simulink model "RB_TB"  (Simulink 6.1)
settings: Solver=ode3  SolverMode=SingleTasking  StartTime=0  StopTime=0.1  FixedStep=0.01  RelTol=1e-3
libraries: simulink x2
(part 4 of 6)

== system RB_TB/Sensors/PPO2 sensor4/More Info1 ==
  note: Terminology:
  note: Sensor fusion by using a sliding observer for an underwater breathing system Salvatore Carotenuto, Luigi Iannelli, Sabato Manfredi, Stefania Santini e-mail: luigi.iannelli@unisannio.it, {salcarot, smanfred, stsantin}@unina.it ... When working in critical conditions or environments, such as under the sea, the control-loop has to be fault-tolerant. In other words the control strategy of the rebreather system has to be 'robust' against sensor failures. An error on the actual oxygen level measurement, especially in the set point proximity, can cause a disease to the diver and may have fatal consequences. Thus, in the counterlung control-loop some hardware redundancy is desired: usually the system output (oxygen partial pressure) is measured through three sensors so that eventual sensor faults can be detected and isolated for the diver safety. Of course, by introducing this redundancy, an algorithm that decides which measurement value to give to the controller is needed. The problem of designing this algorithm is called 'sensor fusion' problem. ... The performance of the proposed strategy are discussed comparing it with a more traditional approach based on a decision by majority criteria [7], [8], usually named as voting logic, which is currently implemented in some commercial rebreathers and is a proven technology in some applicative areas as fly-by-wire control [9].

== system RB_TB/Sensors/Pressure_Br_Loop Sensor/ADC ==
  note: This subsystem models a typical 15-bit analog-to-digital converter having an input range of 0-3 volts
  note: Model: RB_TB/Sensors/Pressure_ambient Sensor/ADC
  voltage : Inport  Port=1  LatchInput=off
  limit : Saturate  UpperLimit=2^15  LowerLimit=0
  quantize : Quantizer  QuantizationInterval=1
  scale : Gain  Gain=2^15/3
  pcm : Outport
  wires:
  voltage/1 -> scale/1
  quantize/1 -> limit/1
  scale/1 -> quantize/1
  limit/1 -> pcm/1

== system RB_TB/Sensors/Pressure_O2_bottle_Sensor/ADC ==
  note: Model: RB_TB/Sensors/Pressure_ambient Sensor/ADC
  note: This subsystem models a typical 15-bit analog-to-digital converter having an input range of 0-3 volts
  voltage : Inport  Port=1  LatchInput=off
  limit : Saturate  UpperLimit=2^15  LowerLimit=0
  quantize : Quantizer  QuantizationInterval=1
  scale : Gain  Gain=2^15/3
  pcm : Outport
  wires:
  limit/1 -> pcm/1
  scale/1 -> quantize/1
  quantize/1 -> limit/1
  voltage/1 -> scale/1

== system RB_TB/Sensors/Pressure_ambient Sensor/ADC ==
  note: Model: RB_TB/Sensors/Pressure_ambient Sensor/ADC
  note: This subsystem models a typical 15-bit analog-to-digital converter having an input range of 0-3 volts
  voltage : Inport  Port=1  LatchInput=off
  limit : Saturate  UpperLimit=2^15  LowerLimit=0
  quantize : Quantizer  QuantizationInterval=1
  scale : Gain  Gain=2^15/3
  pcm : Outport
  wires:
  limit/1 -> pcm/1
  scale/1 -> quantize/1
  quantize/1 -> limit/1
  voltage/1 -> scale/1

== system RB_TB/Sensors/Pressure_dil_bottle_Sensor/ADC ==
  note: This subsystem models a typical 15-bit analog-to-digital converter having an input range of 0-3 volts
  note: Model: RB_TB/Sensors/Pressure_ambient Sensor/ADC
  voltage : Inport  Port=1  LatchInput=off
  limit : Saturate  UpperLimit=2^15  LowerLimit=0
  quantize : Quantizer  QuantizationInterval=1
  scale : Gain  Gain=2^15/3
  pcm : Outport
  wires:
  voltage/1 -> scale/1
  quantize/1 -> limit/1
  scale/1 -> quantize/1
  limit/1 -> pcm/1

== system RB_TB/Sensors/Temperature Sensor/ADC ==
  note: This subsystem models a typical 16-bit analog-to-digital converter having an input range of 0-5 volts
  note: Model: RB_TB/Sensors/temperature_sensor/ADC
  voltage : Inport  Port=1  LatchInput=off
  limit : Saturate  UpperLimit=65535  LowerLimit=0
  quantize : Quantizer  QuantizationInterval=1
  scale : Gain  Gain=65536/5
  pcm : Outport
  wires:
  voltage/1 -> scale/1
  quantize/1 -> limit/1
  scale/1 -> quantize/1
  limit/1 -> pcm/1

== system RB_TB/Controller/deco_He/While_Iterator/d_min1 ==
  note: Model: RB_TB/Controller/deco_He/While_Iterator/d_minX
  Pt_new : Inport  Port=1  LatchInput=off
  In1 : Inport  Port=2  LatchInput=off
  In2 : Inport  Port=3  LatchInput=off
  BC : BusCreator  DialogController=Simulink.DDGSource_Bus
  BS1 : BusSelector  DialogController=Simulink.DDGSource_Bus  OutputSignals=He_b,M0,He_k,Pt
  BS2 : BusSelector  DialogController=Simulink.DDGSource_Bus  OutputSignals=rate_asc,asc_time,while,cnc_He,Palv_next,Palv
  Mux2 : Mux  Inputs=6
  Product2 : Product
  Sum1 : Sum  Inputs=-+|
  Switch : Switch  Threshold=2
  Switch1 : Switch  Threshold=2
  fnc : Fcn  Expr=u(6)-u(5)*u(2)*(u(3)-1/u(1))-(u(6)-u(4)+u(5)*u(2)/u(1))*exp(-u(1)*u(3))
  prod : Gain  Gain=10
  bus1 : Outport
  d_min : Outport  Port=2
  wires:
  BS2/1 -> Mux2/2  "<rate_asc>"
  In2/1 -> BS2/1
  BS2/5 -> Switch1/1  "<Palv_next>"
  BS2/3 -> Switch1/2, Switch/2  "<while>"
  BS2/6 -> Switch1/3  "<Palv>"
  Switch1/1 -> Mux2/6
  Pt_new/1 -> Switch/1
  BS1/4 -> Switch/3  "<Pt>"
  Switch/1 -> Mux2/4, Sum1/2  "Pt"
  BC/1 -> bus1/1
  Product2/1 -> d_min/1
  prod/1 -> Product2/1
  Sum1/1 -> Product2/2
  In1/1 -> BS1/1
  BS2/4 -> Mux2/5  "<cnc_He>"
  BS2/2 -> Mux2/3  "<asc_time>"
  fnc/1 -> BC/4  "Pt_stop"
  Mux2/1 -> fnc/1
  BS1/2 -> BC/2, Sum1/1  "<M0>"
  BS1/1 -> BC/1, prod/1  "<He_b>"
  BS1/3 -> BC/3, Mux2/1  "<He_k>"

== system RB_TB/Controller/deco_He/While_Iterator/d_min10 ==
  note: Model: RB_TB/Controller/deco_He/While_Iterator/d_minX
  Pt_new : Inport  Port=1  LatchInput=off
  In1 : Inport  Port=2  LatchInput=off
  In2 : Inport  Port=3  LatchInput=off
  BC : BusCreator  DialogController=Simulink.DDGSource_Bus
  BS1 : BusSelector  DialogController=Simulink.DDGSource_Bus  OutputSignals=He_b,M0,He_k,Pt
  BS2 : BusSelector  DialogController=Simulink.DDGSource_Bus  OutputSignals=rate_asc,asc_time,while,cnc_He,Palv_next,Palv
  Mux2 : Mux  Inputs=6
  Product2 : Product
  Sum1 : Sum  Inputs=-+|
  Switch : Switch  Threshold=2
  Switch1 : Switch  Threshold=2
  fnc : Fcn  Expr=u(6)-u(5)*u(2)*(u(3)-1/u(1))-(u(6)-u(4)+u(5)*u(2)/u(1))*exp(-u(1)*u(3))
  prod : Gain  Gain=10
  bus1 : Outport
  d_min : Outport  Port=2
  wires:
  BS1/3 -> Mux2/1, BC/3  "<He_k>"
  BS1/1 -> prod/1, BC/1  "<He_b>"
  BS1/2 -> Sum1/1, BC/2  "<M0>"
  Mux2/1 -> fnc/1
  fnc/1 -> BC/4  "Pt_stop"
  BS2/2 -> Mux2/3  "<asc_time>"
  BS2/4 -> Mux2/5  "<cnc_He>"
  In1/1 -> BS1/1
  Sum1/1 -> Product2/2
  prod/1 -> Product2/1
  Product2/1 -> d_min/1
  BC/1 -> bus1/1
  Switch/1 -> Sum1/2, Mux2/4  "Pt"
  BS1/4 -> Switch/3  "<Pt>"
  Pt_new/1 -> Switch/1
  Switch1/1 -> Mux2/6
  BS2/6 -> Switch1/3  "<Palv>"
  BS2/3 -> Switch/2, Switch1/2  "<while>"
  BS2/5 -> Switch1/1  "<Palv_next>"
  In2/1 -> BS2/1
  BS2/1 -> Mux2/2  "<rate_asc>"

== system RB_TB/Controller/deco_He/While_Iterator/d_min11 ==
  note: Model: RB_TB/Controller/deco_He/While_Iterator/d_minX
  Pt_new : Inport  Port=1  LatchInput=off
  In1 : Inport  Port=2  LatchInput=off
  In2 : Inport  Port=3  LatchInput=off
  BC : BusCreator  DialogController=Simulink.DDGSource_Bus
  BS1 : BusSelector  DialogController=Simulink.DDGSource_Bus  OutputSignals=He_b,M0,He_k,Pt
  BS2 : BusSelector  DialogController=Simulink.DDGSource_Bus  OutputSignals=rate_asc,asc_time,while,cnc_He,Palv_next,Palv
  Mux2 : Mux  Inputs=6
  Product2 : Product
  Sum1 : Sum  Inputs=-+|
  Switch : Switch  Threshold=2
  Switch1 : Switch  Threshold=2
  fnc : Fcn  Expr=u(6)-u(5)*u(2)*(u(3)-1/u(1))-(u(6)-u(4)+u(5)*u(2)/u(1))*exp(-u(1)*u(3))
  prod : Gain  Gain=10
  bus1 : Outport
  d_min : Outport  Port=2
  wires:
  BS2/1 -> Mux2/2  "<rate_asc>"
  In2/1 -> BS2/1
  BS2/5 -> Switch1/1  "<Palv_next>"
  BS2/3 -> Switch1/2, Switch/2  "<while>"
  BS2/6 -> Switch1/3  "<Palv>"
  Switch1/1 -> Mux2/6
  Pt_new/1 -> Switch/1
  BS1/4 -> Switch/3  "<Pt>"
  Switch/1 -> Mux2/4, Sum1/2  "Pt"
  BC/1 -> bus1/1
  Product2/1 -> d_min/1
  prod/1 -> Product2/1
  Sum1/1 -> Product2/2
  In1/1 -> BS1/1
  BS2/4 -> Mux2/5  "<cnc_He>"
  BS2/2 -> Mux2/3  "<asc_time>"
  fnc/1 -> BC/4  "Pt_stop"
  Mux2/1 -> fnc/1
  BS1/2 -> BC/2, Sum1/1  "<M0>"
  BS1/1 -> BC/1, prod/1  "<He_b>"
  BS1/3 -> BC/3, Mux2/1  "<He_k>"

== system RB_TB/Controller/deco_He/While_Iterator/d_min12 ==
  note: Model: RB_TB/Controller/deco_He/While_Iterator/d_minX
  Pt_new : Inport  Port=1  LatchInput=off
  In1 : Inport  Port=2  LatchInput=off
  In2 : Inport  Port=3  LatchInput=off
  BC : BusCreator  DialogController=Simulink.DDGSource_Bus
  BS1 : BusSelector  DialogController=Simulink.DDGSource_Bus  OutputSignals=He_b,M0,He_k,Pt
  BS2 : BusSelector  DialogController=Simulink.DDGSource_Bus  OutputSignals=rate_asc,asc_time,while,cnc_He,Palv_next,Palv
  Mux2 : Mux  Inputs=6
  Product2 : Product
  Sum1 : Sum  Inputs=-+|
  Switch : Switch  Threshold=2
  Switch1 : Switch  Threshold=2
  fnc : Fcn  Expr=u(6)-u(5)*u(2)*(u(3)-1/u(1))-(u(6)-u(4)+u(5)*u(2)/u(1))*exp(-u(1)*u(3))
  prod : Gain  Gain=10
  bus1 : Outport
  d_min : Outport  Port=2
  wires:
  BS1/3 -> Mux2/1, BC/3  "<He_k>"
  BS1/1 -> prod/1, BC/1  "<He_b>"
  BS1/2 -> Sum1/1, BC/2  "<M0>"
  Mux2/1 -> fnc/1
  fnc/1 -> BC/4  "Pt_stop"
  BS2/2 -> Mux2/3  "<asc_time>"
  BS2/4 -> Mux2/5  "<cnc_He>"
  In1/1 -> BS1/1
  Sum1/1 -> Product2/2
  prod/1 -> Product2/1
  Product2/1 -> d_min/1
  BC/1 -> bus1/1
  Switch/1 -> Sum1/2, Mux2/4  "Pt"
  BS1/4 -> Switch/3  "<Pt>"
  Pt_new/1 -> Switch/1
  Switch1/1 -> Mux2/6
  BS2/6 -> Switch1/3  "<Palv>"
  BS2/3 -> Switch/2, Switch1/2  "<while>"
  BS2/5 -> Switch1/1  "<Palv_next>"
  In2/1 -> BS2/1
  BS2/1 -> Mux2/2  "<rate_asc>"

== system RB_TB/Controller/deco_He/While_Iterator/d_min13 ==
  note: Model: RB_TB/Controller/deco_He/While_Iterator/d_minX
  Pt_new : Inport  Port=1  LatchInput=off
  In1 : Inport  Port=2  LatchInput=off
  In2 : Inport  Port=3  LatchInput=off
  BC : BusCreator  DialogController=Simulink.DDGSource_Bus
  BS1 : BusSelector  DialogController=Simulink.DDGSource_Bus  OutputSignals=He_b,M0,He_k,Pt
  BS2 : BusSelector  DialogController=Simulink.DDGSource_Bus  OutputSignals=rate_asc,asc_time,while,cnc_He,Palv_next,Palv
  Mux2 : Mux  Inputs=6
  Product2 : Product
  Sum1 : Sum  Inputs=-+|
  Switch : Switch  Threshold=2
  Switch1 : Switch  Threshold=2
  fnc : Fcn  Expr=u(6)-u(5)*u(2)*(u(3)-1/u(1))-(u(6)-u(4)+u(5)*u(2)/u(1))*exp(-u(1)*u(3))
  prod : Gain  Gain=10
  bus1 : Outport
  d_min : Outport  Port=2
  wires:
  BS2/1 -> Mux2/2  "<rate_asc>"
  In2/1 -> BS2/1
  BS2/5 -> Switch1/1  "<Palv_next>"
  BS2/3 -> Switch1/2, Switch/2  "<while>"
  BS2/6 -> Switch1/3  "<Palv>"
  Switch1/1 -> Mux2/6
  Pt_new/1 -> Switch/1
  BS1/4 -> Switch/3  "<Pt>"
  Switch/1 -> Mux2/4, Sum1/2  "Pt"
  BC/1 -> bus1/1
  Product2/1 -> d_min/1
  prod/1 -> Product2/1
  Sum1/1 -> Product2/2
  In1/1 -> BS1/1
  BS2/4 -> Mux2/5  "<cnc_He>"
  BS2/2 -> Mux2/3  "<asc_time>"
  fnc/1 -> BC/4  "Pt_stop"
  Mux2/1 -> fnc/1
  BS1/2 -> BC/2, Sum1/1  "<M0>"
  BS1/1 -> BC/1, prod/1  "<He_b>"
  BS1/3 -> BC/3, Mux2/1  "<He_k>"

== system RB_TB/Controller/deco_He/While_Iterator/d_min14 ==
  note: Model: RB_TB/Controller/deco_He/While_Iterator/d_minX
  Pt_new : Inport  Port=1  LatchInput=off
  In1 : Inport  Port=2  LatchInput=off
  In2 : Inport  Port=3  LatchInput=off
  BC : BusCreator  DialogController=Simulink.DDGSource_Bus
  BS1 : BusSelector  DialogController=Simulink.DDGSource_Bus  OutputSignals=He_b,M0,He_k,Pt
  BS2 : BusSelector  DialogController=Simulink.DDGSource_Bus  OutputSignals=rate_asc,asc_time,while,cnc_He,Palv_next,Palv
  Mux2 : Mux  Inputs=6
  Product2 : Product
  Sum1 : Sum  Inputs=-+|
  Switch : Switch  Threshold=2
  Switch1 : Switch  Threshold=2
  fnc : Fcn  Expr=u(6)-u(5)*u(2)*(u(3)-1/u(1))-(u(6)-u(4)+u(5)*u(2)/u(1))*exp(-u(1)*u(3))
  prod : Gain  Gain=10
  bus1 : Outport
  d_min : Outport  Port=2
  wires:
  BS1/3 -> Mux2/1, BC/3  "<He_k>"
  BS1/1 -> prod/1, BC/1  "<He_b>"
  BS1/2 -> Sum1/1, BC/2  "<M0>"
  Mux2/1 -> fnc/1
  fnc/1 -> BC/4  "Pt_stop"
  BS2/2 -> Mux2/3  "<asc_time>"
  BS2/4 -> Mux2/5  "<cnc_He>"
  In1/1 -> BS1/1
  Sum1/1 -> Product2/2
  prod/1 -> Product2/1
  Product2/1 -> d_min/1
  BC/1 -> bus1/1
  Switch/1 -> Sum1/2, Mux2/4  "Pt"
  BS1/4 -> Switch/3  "<Pt>"
  Pt_new/1 -> Switch/1
  Switch1/1 -> Mux2/6
  BS2/6 -> Switch1/3  "<Palv>"
  BS2/3 -> Switch/2, Switch1/2  "<while>"
  BS2/5 -> Switch1/1  "<Palv_next>"
  In2/1 -> BS2/1
  BS2/1 -> Mux2/2  "<rate_asc>"

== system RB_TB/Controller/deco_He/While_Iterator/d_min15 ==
  note: Model: RB_TB/Controller/deco_He/While_Iterator/d_minX
  Pt_new : Inport  Port=1  LatchInput=off
  In1 : Inport  Port=2  LatchInput=off
  In2 : Inport  Port=3  LatchInput=off
  BC : BusCreator  DialogController=Simulink.DDGSource_Bus
  BS1 : BusSelector  DialogController=Simulink.DDGSource_Bus  OutputSignals=He_b,M0,He_k,Pt
  BS2 : BusSelector  DialogController=Simulink.DDGSource_Bus  OutputSignals=rate_asc,asc_time,while,cnc_He,Palv_next,Palv
  Mux2 : Mux  Inputs=6
  Product2 : Product
  Sum1 : Sum  Inputs=-+|
  Switch : Switch  Threshold=2
  Switch1 : Switch  Threshold=2
  fnc : Fcn  Expr=u(6)-u(5)*u(2)*(u(3)-1/u(1))-(u(6)-u(4)+u(5)*u(2)/u(1))*exp(-u(1)*u(3))
  prod : Gain  Gain=10
  bus1 : Outport
  d_min : Outport  Port=2
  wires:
  BS2/1 -> Mux2/2  "<rate_asc>"
  In2/1 -> BS2/1
  BS2/5 -> Switch1/1  "<Palv_next>"
  BS2/3 -> Switch1/2, Switch/2  "<while>"
  BS2/6 -> Switch1/3  "<Palv>"
  Switch1/1 -> Mux2/6
  Pt_new/1 -> Switch/1
  BS1/4 -> Switch/3  "<Pt>"
  Switch/1 -> Mux2/4, Sum1/2  "Pt"
  BC/1 -> bus1/1
  Product2/1 -> d_min/1
  prod/1 -> Product2/1
  Sum1/1 -> Product2/2
  In1/1 -> BS1/1
  BS2/4 -> Mux2/5  "<cnc_He>"
  BS2/2 -> Mux2/3  "<asc_time>"
  fnc/1 -> BC/4  "Pt_stop"
  Mux2/1 -> fnc/1
  BS1/2 -> BC/2, Sum1/1  "<M0>"
  BS1/1 -> BC/1, prod/1  "<He_b>"
  BS1/3 -> BC/3, Mux2/1  "<He_k>"

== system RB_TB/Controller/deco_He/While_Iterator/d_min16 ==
  note: Model: RB_TB/Controller/deco_He/While_Iterator/d_minX
  Pt_new : Inport  Port=1  LatchInput=off
  In1 : Inport  Port=2  LatchInput=off
  In2 : Inport  Port=3  LatchInput=off
  BC : BusCreator  DialogController=Simulink.DDGSource_Bus
  BS1 : BusSelector  DialogController=Simulink.DDGSource_Bus  OutputSignals=He_b,M0,He_k,Pt
  BS2 : BusSelector  DialogController=Simulink.DDGSource_Bus  OutputSignals=rate_asc,asc_time,while,cnc_He,Palv_next,Palv
  Mux2 : Mux  Inputs=6
  Product2 : Product
  Sum1 : Sum  Inputs=-+|
  Switch : Switch  Threshold=2
  Switch1 : Switch  Threshold=2
  fnc : Fcn  Expr=u(6)-u(5)*u(2)*(u(3)-1/u(1))-(u(6)-u(4)+u(5)*u(2)/u(1))*exp(-u(1)*u(3))
  prod : Gain  Gain=10
  bus1 : Outport
  d_min : Outport  Port=2
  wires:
  BS1/3 -> Mux2/1, BC/3  "<He_k>"
  BS1/1 -> prod/1, BC/1  "<He_b>"
  BS1/2 -> Sum1/1, BC/2  "<M0>"
  Mux2/1 -> fnc/1
  fnc/1 -> BC/4  "Pt_stop"
  BS2/2 -> Mux2/3  "<asc_time>"
  BS2/4 -> Mux2/5  "<cnc_He>"
  In1/1 -> BS1/1
  Sum1/1 -> Product2/2
  prod/1 -> Product2/1
  Product2/1 -> d_min/1
  BC/1 -> bus1/1
  Switch/1 -> Sum1/2, Mux2/4  "Pt"
  BS1/4 -> Switch/3  "<Pt>"
  Pt_new/1 -> Switch/1
  Switch1/1 -> Mux2/6
  BS2/6 -> Switch1/3  "<Palv>"
  BS2/3 -> Switch/2, Switch1/2  "<while>"
  BS2/5 -> Switch1/1  "<Palv_next>"
  In2/1 -> BS2/1
  BS2/1 -> Mux2/2  "<rate_asc>"

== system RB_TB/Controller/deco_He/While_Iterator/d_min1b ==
  note: Model: RB_TB/Controller/deco_He/While_Iterator/d_minX
  Pt_new : Inport  Port=1  LatchInput=off
  In1 : Inport  Port=2  LatchInput=off
  In2 : Inport  Port=3  LatchInput=off
  BC : BusCreator  DialogController=Simulink.DDGSource_Bus
  BS1 : BusSelector  DialogController=Simulink.DDGSource_Bus  OutputSignals=He_b,M0,He_k,Pt
  BS2 : BusSelector  DialogController=Simulink.DDGSource_Bus  OutputSignals=rate_asc,asc_time,while,cnc_He,Palv_next,Palv
  Mux2 : Mux  Inputs=6
  Product2 : Product
  Sum1 : Sum  Inputs=-+|
  Switch : Switch  Threshold=2
  Switch1 : Switch  Threshold=2
  fnc : Fcn  Expr=u(6)-u(5)*u(2)*(u(3)-1/u(1))-(u(6)-u(4)+u(5)*u(2)/u(1))*exp(-u(1)*u(3))
  prod : Gain  Gain=10
  bus1 : Outport
  d_min : Outport  Port=2
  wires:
  BS2/1 -> Mux2/2  "<rate_asc>"
  In2/1 -> BS2/1
  BS2/5 -> Switch1/1  "<Palv_next>"
  BS2/3 -> Switch1/2, Switch/2  "<while>"
  BS2/6 -> Switch1/3  "<Palv>"
  Switch1/1 -> Mux2/6
  Pt_new/1 -> Switch/1
  BS1/4 -> Switch/3  "<Pt>"
  Switch/1 -> Mux2/4, Sum1/2  "Pt"
  BC/1 -> bus1/1
  Product2/1 -> d_min/1
  prod/1 -> Product2/1
  Sum1/1 -> Product2/2
  In1/1 -> BS1/1
  BS2/4 -> Mux2/5  "<cnc_He>"
  BS2/2 -> Mux2/3  "<asc_time>"
  fnc/1 -> BC/4  "Pt_stop"
  Mux2/1 -> fnc/1
  BS1/2 -> BC/2, Sum1/1  "<M0>"
  BS1/1 -> BC/1, prod/1  "<He_b>"
  BS1/3 -> BC/3, Mux2/1  "<He_k>"

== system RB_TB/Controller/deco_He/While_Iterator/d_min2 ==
  note: Model: RB_TB/Controller/deco_He/While_Iterator/d_minX
  Pt_new : Inport  Port=1  LatchInput=off
  In1 : Inport  Port=2  LatchInput=off
  In2 : Inport  Port=3  LatchInput=off
  BC : BusCreator  DialogController=Simulink.DDGSource_Bus
  BS1 : BusSelector  DialogController=Simulink.DDGSource_Bus  OutputSignals=He_b,M0,He_k,Pt
  BS2 : BusSelector  DialogController=Simulink.DDGSource_Bus  OutputSignals=rate_asc,asc_time,while,cnc_He,Palv_next,Palv
  Mux2 : Mux  Inputs=6
  Product2 : Product
  Sum1 : Sum  Inputs=-+|
  Switch : Switch  Threshold=2
  Switch1 : Switch  Threshold=2
  fnc : Fcn  Expr=u(6)-u(5)*u(2)*(u(3)-1/u(1))-(u(6)-u(4)+u(5)*u(2)/u(1))*exp(-u(1)*u(3))
  prod : Gain  Gain=10
  bus1 : Outport
  d_min : Outport  Port=2
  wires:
  BS1/3 -> Mux2/1, BC/3  "<He_k>"
  BS1/1 -> prod/1, BC/1  "<He_b>"
  BS1/2 -> Sum1/1, BC/2  "<M0>"
  Mux2/1 -> fnc/1
  fnc/1 -> BC/4  "Pt_stop"
  BS2/2 -> Mux2/3  "<asc_time>"
  BS2/4 -> Mux2/5  "<cnc_He>"
  In1/1 -> BS1/1
  Sum1/1 -> Product2/2
  prod/1 -> Product2/1
  Product2/1 -> d_min/1
  BC/1 -> bus1/1
  Switch/1 -> Sum1/2, Mux2/4  "Pt"
  BS1/4 -> Switch/3  "<Pt>"
  Pt_new/1 -> Switch/1
  Switch1/1 -> Mux2/6
  BS2/6 -> Switch1/3  "<Palv>"
  BS2/3 -> Switch/2, Switch1/2  "<while>"
  BS2/5 -> Switch1/1  "<Palv_next>"
  In2/1 -> BS2/1
  BS2/1 -> Mux2/2  "<rate_asc>"

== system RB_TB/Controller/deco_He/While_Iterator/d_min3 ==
  note: Model: RB_TB/Controller/deco_He/While_Iterator/d_minX
  Pt_new : Inport  Port=1  LatchInput=off
  In1 : Inport  Port=2  LatchInput=off
  In2 : Inport  Port=3  LatchInput=off
  BC : BusCreator  DialogController=Simulink.DDGSource_Bus
  BS1 : BusSelector  DialogController=Simulink.DDGSource_Bus  OutputSignals=He_b,M0,He_k,Pt
  BS2 : BusSelector  DialogController=Simulink.DDGSource_Bus  OutputSignals=rate_asc,asc_time,while,cnc_He,Palv_next,Palv
  Mux2 : Mux  Inputs=6
  Product2 : Product
  Sum1 : Sum  Inputs=-+|
  Switch : Switch  Threshold=2
  Switch1 : Switch  Threshold=2
  fnc : Fcn  Expr=u(6)-u(5)*u(2)*(u(3)-1/u(1))-(u(6)-u(4)+u(5)*u(2)/u(1))*exp(-u(1)*u(3))
  prod : Gain  Gain=10
  bus1 : Outport
  d_min : Outport  Port=2
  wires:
  BS2/1 -> Mux2/2  "<rate_asc>"
  In2/1 -> BS2/1
  BS2/5 -> Switch1/1  "<Palv_next>"
  BS2/3 -> Switch1/2, Switch/2  "<while>"
  BS2/6 -> Switch1/3  "<Palv>"
  Switch1/1 -> Mux2/6
  Pt_new/1 -> Switch/1
  BS1/4 -> Switch/3  "<Pt>"
  Switch/1 -> Mux2/4, Sum1/2  "Pt"
  BC/1 -> bus1/1
  Product2/1 -> d_min/1
  prod/1 -> Product2/1
  Sum1/1 -> Product2/2
  In1/1 -> BS1/1
  BS2/4 -> Mux2/5  "<cnc_He>"
  BS2/2 -> Mux2/3  "<asc_time>"
  fnc/1 -> BC/4  "Pt_stop"
  Mux2/1 -> fnc/1
  BS1/2 -> BC/2, Sum1/1  "<M0>"
  BS1/1 -> BC/1, prod/1  "<He_b>"
  BS1/3 -> BC/3, Mux2/1  "<He_k>"

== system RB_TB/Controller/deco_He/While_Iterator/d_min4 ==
  note: Model: RB_TB/Controller/deco_He/While_Iterator/d_minX
  Pt_new : Inport  Port=1  LatchInput=off
  In1 : Inport  Port=2  LatchInput=off
  In2 : Inport  Port=3  LatchInput=off
  BC : BusCreator  DialogController=Simulink.DDGSource_Bus
  BS1 : BusSelector  DialogController=Simulink.DDGSource_Bus  OutputSignals=He_b,M0,He_k,Pt
  BS2 : BusSelector  DialogController=Simulink.DDGSource_Bus  OutputSignals=rate_asc,asc_time,while,cnc_He,Palv_next,Palv
  Mux2 : Mux  Inputs=6
  Product2 : Product
  Sum1 : Sum  Inputs=-+|
  Switch : Switch  Threshold=2
  Switch1 : Switch  Threshold=2
  fnc : Fcn  Expr=u(6)-u(5)*u(2)*(u(3)-1/u(1))-(u(6)-u(4)+u(5)*u(2)/u(1))*exp(-u(1)*u(3))
  prod : Gain  Gain=10
  bus1 : Outport
  d_min : Outport  Port=2
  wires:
  BS1/3 -> Mux2/1, BC/3  "<He_k>"
  BS1/1 -> prod/1, BC/1  "<He_b>"
  BS1/2 -> Sum1/1, BC/2  "<M0>"
  Mux2/1 -> fnc/1
  fnc/1 -> BC/4  "Pt_stop"
  BS2/2 -> Mux2/3  "<asc_time>"
  BS2/4 -> Mux2/5  "<cnc_He>"
  In1/1 -> BS1/1
  Sum1/1 -> Product2/2
  prod/1 -> Product2/1
  Product2/1 -> d_min/1
  BC/1 -> bus1/1
  Switch/1 -> Sum1/2, Mux2/4  "Pt"
  BS1/4 -> Switch/3  "<Pt>"
  Pt_new/1 -> Switch/1
  Switch1/1 -> Mux2/6
  BS2/6 -> Switch1/3  "<Palv>"
  BS2/3 -> Switch/2, Switch1/2  "<while>"
  BS2/5 -> Switch1/1  "<Palv_next>"
  In2/1 -> BS2/1
  BS2/1 -> Mux2/2  "<rate_asc>"

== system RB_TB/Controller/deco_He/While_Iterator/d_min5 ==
  note: Model: RB_TB/Controller/deco_He/While_Iterator/d_minX
  Pt_new : Inport  Port=1  LatchInput=off
  In1 : Inport  Port=2  LatchInput=off
  In2 : Inport  Port=3  LatchInput=off
  BC : BusCreator  DialogController=Simulink.DDGSource_Bus
  BS1 : BusSelector  DialogController=Simulink.DDGSource_Bus  OutputSignals=He_b,M0,He_k,Pt
  BS2 : BusSelector  DialogController=Simulink.DDGSource_Bus  OutputSignals=rate_asc,asc_time,while,cnc_He,Palv_next,Palv
  Mux2 : Mux  Inputs=6
  Product2 : Product
  Sum1 : Sum  Inputs=-+|
  Switch : Switch  Threshold=2
  Switch1 : Switch  Threshold=2
  fnc : Fcn  Expr=u(6)-u(5)*u(2)*(u(3)-1/u(1))-(u(6)-u(4)+u(5)*u(2)/u(1))*exp(-u(1)*u(3))
  prod : Gain  Gain=10
  bus1 : Outport
  d_min : Outport  Port=2
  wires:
  BS2/1 -> Mux2/2  "<rate_asc>"
  In2/1 -> BS2/1
  BS2/5 -> Switch1/1  "<Palv_next>"
  BS2/3 -> Switch1/2, Switch/2  "<while>"
  BS2/6 -> Switch1/3  "<Palv>"
  Switch1/1 -> Mux2/6
  Pt_new/1 -> Switch/1
  BS1/4 -> Switch/3  "<Pt>"
  Switch/1 -> Mux2/4, Sum1/2  "Pt"
  BC/1 -> bus1/1
  Product2/1 -> d_min/1
  prod/1 -> Product2/1
  Sum1/1 -> Product2/2
  In1/1 -> BS1/1
  BS2/4 -> Mux2/5  "<cnc_He>"
  BS2/2 -> Mux2/3  "<asc_time>"
  fnc/1 -> BC/4  "Pt_stop"
  Mux2/1 -> fnc/1
  BS1/2 -> BC/2, Sum1/1  "<M0>"
  BS1/1 -> BC/1, prod/1  "<He_b>"
  BS1/3 -> BC/3, Mux2/1  "<He_k>"

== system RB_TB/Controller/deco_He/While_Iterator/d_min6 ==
  note: Model: RB_TB/Controller/deco_He/While_Iterator/d_minX
  Pt_new : Inport  Port=1  LatchInput=off
  In1 : Inport  Port=2  LatchInput=off
  In2 : Inport  Port=3  LatchInput=off
  BC : BusCreator  DialogController=Simulink.DDGSource_Bus
  BS1 : BusSelector  DialogController=Simulink.DDGSource_Bus  OutputSignals=He_b,M0,He_k,Pt
  BS2 : BusSelector  DialogController=Simulink.DDGSource_Bus  OutputSignals=rate_asc,asc_time,while,cnc_He,Palv_next,Palv
  Mux2 : Mux  Inputs=6
  Product2 : Product
  Sum1 : Sum  Inputs=-+|
  Switch : Switch  Threshold=2
  Switch1 : Switch  Threshold=2
  fnc : Fcn  Expr=u(6)-u(5)*u(2)*(u(3)-1/u(1))-(u(6)-u(4)+u(5)*u(2)/u(1))*exp(-u(1)*u(3))
  prod : Gain  Gain=10
  bus1 : Outport
  d_min : Outport  Port=2
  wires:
  BS1/3 -> Mux2/1, BC/3  "<He_k>"
  BS1/1 -> prod/1, BC/1  "<He_b>"
  BS1/2 -> Sum1/1, BC/2  "<M0>"
  Mux2/1 -> fnc/1
  fnc/1 -> BC/4  "Pt_stop"
  BS2/2 -> Mux2/3  "<asc_time>"
  BS2/4 -> Mux2/5  "<cnc_He>"
  In1/1 -> BS1/1
  Sum1/1 -> Product2/2
  prod/1 -> Product2/1
  Product2/1 -> d_min/1
  BC/1 -> bus1/1
  Switch/1 -> Sum1/2, Mux2/4  "Pt"
  BS1/4 -> Switch/3  "<Pt>"
  Pt_new/1 -> Switch/1
  Switch1/1 -> Mux2/6
  BS2/6 -> Switch1/3  "<Palv>"
  BS2/3 -> Switch/2, Switch1/2  "<while>"
  BS2/5 -> Switch1/1  "<Palv_next>"
  In2/1 -> BS2/1
  BS2/1 -> Mux2/2  "<rate_asc>"

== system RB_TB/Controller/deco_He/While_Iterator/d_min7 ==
  note: Model: RB_TB/Controller/deco_He/While_Iterator/d_minX
  Pt_new : Inport  Port=1  LatchInput=off
  In1 : Inport  Port=2  LatchInput=off
  In2 : Inport  Port=3  LatchInput=off
  BC : BusCreator  DialogController=Simulink.DDGSource_Bus
  BS1 : BusSelector  DialogController=Simulink.DDGSource_Bus  OutputSignals=He_b,M0,He_k,Pt
  BS2 : BusSelector  DialogController=Simulink.DDGSource_Bus  OutputSignals=rate_asc,asc_time,while,cnc_He,Palv_next,Palv
  Mux2 : Mux  Inputs=6
  Product2 : Product
  Sum1 : Sum  Inputs=-+|
  Switch : Switch  Threshold=2
  Switch1 : Switch  Threshold=2
  fnc : Fcn  Expr=u(6)-u(5)*u(2)*(u(3)-1/u(1))-(u(6)-u(4)+u(5)*u(2)/u(1))*exp(-u(1)*u(3))
  prod : Gain  Gain=10
  bus1 : Outport
  d_min : Outport  Port=2
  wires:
  BS2/1 -> Mux2/2  "<rate_asc>"
  In2/1 -> BS2/1
  BS2/5 -> Switch1/1  "<Palv_next>"
  BS2/3 -> Switch1/2, Switch/2  "<while>"
  BS2/6 -> Switch1/3  "<Palv>"
  Switch1/1 -> Mux2/6
  Pt_new/1 -> Switch/1
  BS1/4 -> Switch/3  "<Pt>"
  Switch/1 -> Mux2/4, Sum1/2  "Pt"
  BC/1 -> bus1/1
  Product2/1 -> d_min/1
  prod/1 -> Product2/1
  Sum1/1 -> Product2/2
  In1/1 -> BS1/1
  BS2/4 -> Mux2/5  "<cnc_He>"
  BS2/2 -> Mux2/3  "<asc_time>"
  fnc/1 -> BC/4  "Pt_stop"
  Mux2/1 -> fnc/1
  BS1/2 -> BC/2, Sum1/1  "<M0>"
  BS1/1 -> BC/1, prod/1  "<He_b>"
  BS1/3 -> BC/3, Mux2/1  "<He_k>"

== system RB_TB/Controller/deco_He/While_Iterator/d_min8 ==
  note: Model: RB_TB/Controller/deco_He/While_Iterator/d_minX
  Pt_new : Inport  Port=1  LatchInput=off
  In1 : Inport  Port=2  LatchInput=off
  In2 : Inport  Port=3  LatchInput=off
  BC : BusCreator  DialogController=Simulink.DDGSource_Bus
  BS1 : BusSelector  DialogController=Simulink.DDGSource_Bus  OutputSignals=He_b,M0,He_k,Pt
  BS2 : BusSelector  DialogController=Simulink.DDGSource_Bus  OutputSignals=rate_asc,asc_time,while,cnc_He,Palv_next,Palv
  Mux2 : Mux  Inputs=6
  Product2 : Product
  Sum1 : Sum  Inputs=-+|
  Switch : Switch  Threshold=2
  Switch1 : Switch  Threshold=2
  fnc : Fcn  Expr=u(6)-u(5)*u(2)*(u(3)-1/u(1))-(u(6)-u(4)+u(5)*u(2)/u(1))*exp(-u(1)*u(3))
  prod : Gain  Gain=10
  bus1 : Outport
  d_min : Outport  Port=2
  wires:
  BS1/3 -> Mux2/1, BC/3  "<He_k>"
  BS1/1 -> prod/1, BC/1  "<He_b>"
  BS1/2 -> Sum1/1, BC/2  "<M0>"
  Mux2/1 -> fnc/1
  fnc/1 -> BC/4  "Pt_stop"
  BS2/2 -> Mux2/3  "<asc_time>"
  BS2/4 -> Mux2/5  "<cnc_He>"
  In1/1 -> BS1/1
  Sum1/1 -> Product2/2
  prod/1 -> Product2/1
  Product2/1 -> d_min/1
  BC/1 -> bus1/1
  Switch/1 -> Sum1/2, Mux2/4  "Pt"
  BS1/4 -> Switch/3  "<Pt>"
  Pt_new/1 -> Switch/1
  Switch1/1 -> Mux2/6
  BS2/6 -> Switch1/3  "<Palv>"
  BS2/3 -> Switch/2, Switch1/2  "<while>"
  BS2/5 -> Switch1/1  "<Palv_next>"
  In2/1 -> BS2/1
  BS2/1 -> Mux2/2  "<rate_asc>"

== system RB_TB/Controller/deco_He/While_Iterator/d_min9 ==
  note: Model: RB_TB/Controller/deco_He/While_Iterator/d_minX
  Pt_new : Inport  Port=1  LatchInput=off
  In1 : Inport  Port=2  LatchInput=off
  In2 : Inport  Port=3  LatchInput=off
  BC : BusCreator  DialogController=Simulink.DDGSource_Bus
  BS1 : BusSelector  DialogController=Simulink.DDGSource_Bus  OutputSignals=He_b,M0,He_k,Pt
  BS2 : BusSelector  DialogController=Simulink.DDGSource_Bus  OutputSignals=rate_asc,asc_time,while,cnc_He,Palv_next,Palv
  Mux2 : Mux  Inputs=6
  Product2 : Product
  Sum1 : Sum  Inputs=-+|
  Switch : Switch  Threshold=2
  Switch1 : Switch  Threshold=2
  fnc : Fcn  Expr=u(6)-u(5)*u(2)*(u(3)-1/u(1))-(u(6)-u(4)+u(5)*u(2)/u(1))*exp(-u(1)*u(3))
  prod : Gain  Gain=10
  bus1 : Outport
  d_min : Outport  Port=2
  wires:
  BS2/1 -> Mux2/2  "<rate_asc>"
  In2/1 -> BS2/1
  BS2/5 -> Switch1/1  "<Palv_next>"
  BS2/3 -> Switch1/2, Switch/2  "<while>"
  BS2/6 -> Switch1/3  "<Palv>"
  Switch1/1 -> Mux2/6
  Pt_new/1 -> Switch/1
  BS1/4 -> Switch/3  "<Pt>"
  Switch/1 -> Mux2/4, Sum1/2  "Pt"
  BC/1 -> bus1/1
  Product2/1 -> d_min/1
  prod/1 -> Product2/1
  Sum1/1 -> Product2/2
  In1/1 -> BS1/1
  BS2/4 -> Mux2/5  "<cnc_He>"
  BS2/2 -> Mux2/3  "<asc_time>"
  fnc/1 -> BC/4  "Pt_stop"
  Mux2/1 -> fnc/1
  BS1/2 -> BC/2, Sum1/1  "<M0>"
  BS1/1 -> BC/1, prod/1  "<He_b>"
  BS1/3 -> BC/3, Mux2/1  "<He_k>"

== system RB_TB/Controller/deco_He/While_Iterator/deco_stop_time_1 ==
  note: Model: RB_TB/Controller/deco_He/While_Iterator/deco_stop_time_X
  In1 : Inport  Port=1  LatchInput=off
  In2 : Inport  Port=2  LatchInput=off
  >10e-300 : Saturate  UpperLimit=inf  LowerLimit=10e-320
  >10e-320 : Switch  Threshold=10e-320
  BS1 : BusSelector  DialogController=Simulink.DDGSource_Bus  OutputSignals=He_k,Pt_stop,He_b,M0
  BS2 : BusSelector  DialogController=Simulink.DDGSource_Bus  OutputSignals=Pstop_next,Palv_next,stop_time
  Constant : Constant
  Mem : Memory  InheritSampleTime=on
  Mux1 : Mux  Inputs=2
  Mux2 : Mux
  Mux3 : Mux  Inputs=2
  Mux4 : Mux  Inputs=3
  Mux5 : Mux  Inputs=3
  fcn(14)1 : Fcn  Expr=log(u(1))
  fcn(14)2 : Fcn  Expr=u(1)-u(2)
  fcn(14)4 : Fcn  Expr=(u(2)-u(3))/u(1)
  fcn(14)5 : Fcn  Expr=-u(2)/u(1)
  fcn1 : Fcn  Expr=u(2)+u(3)/u(1)
  fcn2 : Fcn  Expr=u(3)+(u(2)-u(3))*exp(-u(1)*u(4))
  Pt_new : Outport
  deco_stop_time : Outport  Port=2
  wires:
  >10e-300/1 -> Mux5/1
  Mux5/1 -> fcn(14)4/1
  fcn(14)2/1 -> >10e-300/1
  Mux3/1 -> fcn(14)2/1
  BS2/1 -> Mux4/3  "<Pstop_next>"
  Constant/1 -> >10e-320/3
  fcn(14)4/1 -> >10e-320/1, >10e-320/2
  fcn(14)1/1 -> Mux1/2
  >10e-320/1 -> fcn(14)1/1
  Mux4/1 -> fcn1/1
  fcn(14)5/1 -> deco_stop_time/1  "deco_stop_time"
  fcn1/1 -> Mux5/2  "M_next"
  BS2/2 -> Mux3/2, Mux5/3, Mux2/3  "<Palv_next>"
  BS1/1 -> Mux1/1, Mux2/1  "<He_k>"
  Mux1/1 -> fcn(14)5/1
  BS1/4 -> Mux4/2  "<M0>"
  BS1/3 -> Mux4/1  "<He_b>"
  In1/1 -> BS1/1
  BS1/2 -> Mux3/1, Mux2/2  "<Pt_stop>"
  Mux2/1 -> fcn2/1
  fcn2/1 -> Mem/1
  BS2/3 -> Mux2/4  "<stop_time>"
  Mem/1 -> Pt_new/1
  In2/1 -> BS2/1

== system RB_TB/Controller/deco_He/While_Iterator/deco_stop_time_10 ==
  note: Model: RB_TB/Controller/deco_He/While_Iterator/deco_stop_time_X
  In1 : Inport  Port=1  LatchInput=off
  In2 : Inport  Port=2  LatchInput=off
  >10e-300 : Saturate  UpperLimit=inf  LowerLimit=10e-320
  >10e-320 : Switch  Threshold=10e-320
  BS1 : BusSelector  DialogController=Simulink.DDGSource_Bus  OutputSignals=He_k,Pt_stop,He_b,M0
  BS2 : BusSelector  DialogController=Simulink.DDGSource_Bus  OutputSignals=Pstop_next,Palv_next,stop_time
  Constant : Constant
  Mem : Memory  InheritSampleTime=on
  Mux1 : Mux  Inputs=2
  Mux2 : Mux
  Mux3 : Mux  Inputs=2
  Mux4 : Mux  Inputs=3
  Mux5 : Mux  Inputs=3
  fcn(14)1 : Fcn  Expr=log(u(1))
  fcn(14)2 : Fcn  Expr=u(1)-u(2)
  fcn(14)4 : Fcn  Expr=(u(2)-u(3))/u(1)
  fcn(14)5 : Fcn  Expr=-u(2)/u(1)
  fcn1 : Fcn  Expr=u(2)+u(3)/u(1)
  fcn2 : Fcn  Expr=u(3)+(u(2)-u(3))*exp(-u(1)*u(4))
  Pt_new : Outport
  deco_stop_time : Outport  Port=2
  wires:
  >10e-300/1 -> Mux5/1
  Mux5/1 -> fcn(14)4/1
  fcn(14)2/1 -> >10e-300/1
  Mux3/1 -> fcn(14)2/1
  BS2/1 -> Mux4/3  "<Pstop_next>"
  Constant/1 -> >10e-320/3
  fcn(14)4/1 -> >10e-320/1, >10e-320/2
  fcn(14)1/1 -> Mux1/2
  >10e-320/1 -> fcn(14)1/1
  Mux4/1 -> fcn1/1
  fcn(14)5/1 -> deco_stop_time/1  "deco_stop_time"
  fcn1/1 -> Mux5/2  "M_next"
  BS2/2 -> Mux3/2, Mux5/3, Mux2/3  "<Palv_next>"
  BS1/1 -> Mux1/1, Mux2/1  "<He_k>"
  Mux1/1 -> fcn(14)5/1
  BS1/4 -> Mux4/2  "<M0>"
  BS1/3 -> Mux4/1  "<He_b>"
  In1/1 -> BS1/1
  BS1/2 -> Mux3/1, Mux2/2  "<Pt_stop>"
  Mux2/1 -> fcn2/1
  fcn2/1 -> Mem/1
  BS2/3 -> Mux2/4  "<stop_time>"
  Mem/1 -> Pt_new/1
  In2/1 -> BS2/1

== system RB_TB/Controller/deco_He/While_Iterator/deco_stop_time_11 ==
  note: Model: RB_TB/Controller/deco_He/While_Iterator/deco_stop_time_X
  In1 : Inport  Port=1  LatchInput=off
  In2 : Inport  Port=2  LatchInput=off
  >10e-300 : Saturate  UpperLimit=inf  LowerLimit=10e-320
  >10e-320 : Switch  Threshold=10e-320
  BS1 : BusSelector  DialogController=Simulink.DDGSource_Bus  OutputSignals=He_k,Pt_stop,He_b,M0
  BS2 : BusSelector  DialogController=Simulink.DDGSource_Bus  OutputSignals=Pstop_next,Palv_next,stop_time
  Constant : Constant
  Mem : Memory  InheritSampleTime=on
  Mux1 : Mux  Inputs=2
  Mux2 : Mux
  Mux3 : Mux  Inputs=2
  Mux4 : Mux  Inputs=3
  Mux5 : Mux  Inputs=3
  fcn(14)1 : Fcn  Expr=log(u(1))
  fcn(14)2 : Fcn  Expr=u(1)-u(2)
  fcn(14)4 : Fcn  Expr=(u(2)-u(3))/u(1)
  fcn(14)5 : Fcn  Expr=-u(2)/u(1)
  fcn1 : Fcn  Expr=u(2)+u(3)/u(1)
  fcn2 : Fcn  Expr=u(3)+(u(2)-u(3))*exp(-u(1)*u(4))
  Pt_new : Outport
  deco_stop_time : Outport  Port=2
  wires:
  In2/1 -> BS2/1
  Mem/1 -> Pt_new/1
  BS2/3 -> Mux2/4  "<stop_time>"
  fcn2/1 -> Mem/1
  Mux2/1 -> fcn2/1
  BS1/2 -> Mux2/2, Mux3/1  "<Pt_stop>"
  In1/1 -> BS1/1
  BS1/3 -> Mux4/1  "<He_b>"
  BS1/4 -> Mux4/2  "<M0>"
  Mux1/1 -> fcn(14)5/1
  BS1/1 -> Mux2/1, Mux1/1  "<He_k>"
  BS2/2 -> Mux2/3, Mux5/3, Mux3/2  "<Palv_next>"
  fcn1/1 -> Mux5/2  "M_next"
  fcn(14)5/1 -> deco_stop_time/1  "deco_stop_time"
  Mux4/1 -> fcn1/1
  >10e-320/1 -> fcn(14)1/1
  fcn(14)1/1 -> Mux1/2
  fcn(14)4/1 -> >10e-320/2, >10e-320/1
  Constant/1 -> >10e-320/3
  BS2/1 -> Mux4/3  "<Pstop_next>"
  Mux3/1 -> fcn(14)2/1
  fcn(14)2/1 -> >10e-300/1
  Mux5/1 -> fcn(14)4/1
  >10e-300/1 -> Mux5/1

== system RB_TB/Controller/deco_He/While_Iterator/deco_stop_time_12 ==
  note: Model: RB_TB/Controller/deco_He/While_Iterator/deco_stop_time_X
  In1 : Inport  Port=1  LatchInput=off
  In2 : Inport  Port=2  LatchInput=off
  >10e-300 : Saturate  UpperLimit=inf  LowerLimit=10e-320
  >10e-320 : Switch  Threshold=10e-320
  BS1 : BusSelector  DialogController=Simulink.DDGSource_Bus  OutputSignals=He_k,Pt_stop,He_b,M0
  BS2 : BusSelector  DialogController=Simulink.DDGSource_Bus  OutputSignals=Pstop_next,Palv_next,stop_time
  Constant : Constant
  Mem : Memory  InheritSampleTime=on
  Mux1 : Mux  Inputs=2
  Mux2 : Mux
  Mux3 : Mux  Inputs=2
  Mux4 : Mux  Inputs=3
  Mux5 : Mux  Inputs=3
  fcn(14)1 : Fcn  Expr=log(u(1))
  fcn(14)2 : Fcn  Expr=u(1)-u(2)
  fcn(14)4 : Fcn  Expr=(u(2)-u(3))/u(1)
  fcn(14)5 : Fcn  Expr=-u(2)/u(1)
  fcn1 : Fcn  Expr=u(2)+u(3)/u(1)
  fcn2 : Fcn  Expr=u(3)+(u(2)-u(3))*exp(-u(1)*u(4))
  Pt_new : Outport
  deco_stop_time : Outport  Port=2
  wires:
  >10e-300/1 -> Mux5/1
  Mux5/1 -> fcn(14)4/1
  fcn(14)2/1 -> >10e-300/1
  Mux3/1 -> fcn(14)2/1
  BS2/1 -> Mux4/3  "<Pstop_next>"
  Constant/1 -> >10e-320/3
  fcn(14)4/1 -> >10e-320/1, >10e-320/2
  fcn(14)1/1 -> Mux1/2
  >10e-320/1 -> fcn(14)1/1
  Mux4/1 -> fcn1/1
  fcn(14)5/1 -> deco_stop_time/1  "deco_stop_time"
  fcn1/1 -> Mux5/2  "M_next"
  BS2/2 -> Mux3/2, Mux5/3, Mux2/3  "<Palv_next>"
  BS1/1 -> Mux1/1, Mux2/1  "<He_k>"
  Mux1/1 -> fcn(14)5/1
  BS1/4 -> Mux4/2  "<M0>"
  BS1/3 -> Mux4/1  "<He_b>"
  In1/1 -> BS1/1
  BS1/2 -> Mux3/1, Mux2/2  "<Pt_stop>"
  Mux2/1 -> fcn2/1
  fcn2/1 -> Mem/1
  BS2/3 -> Mux2/4  "<stop_time>"
  Mem/1 -> Pt_new/1
  In2/1 -> BS2/1

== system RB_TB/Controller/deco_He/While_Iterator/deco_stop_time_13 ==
  note: Model: RB_TB/Controller/deco_He/While_Iterator/deco_stop_time_X
  In1 : Inport  Port=1  LatchInput=off
  In2 : Inport  Port=2  LatchInput=off
  >10e-300 : Saturate  UpperLimit=inf  LowerLimit=10e-320
  >10e-320 : Switch  Threshold=10e-320
  BS1 : BusSelector  DialogController=Simulink.DDGSource_Bus  OutputSignals=He_k,Pt_stop,He_b,M0
  BS2 : BusSelector  DialogController=Simulink.DDGSource_Bus  OutputSignals=Pstop_next,Palv_next,stop_time
  Constant : Constant
  Mem : Memory  InheritSampleTime=on
  Mux1 : Mux  Inputs=2
  Mux2 : Mux
  Mux3 : Mux  Inputs=2
  Mux4 : Mux  Inputs=3
  Mux5 : Mux  Inputs=3
  fcn(14)1 : Fcn  Expr=log(u(1))
  fcn(14)2 : Fcn  Expr=u(1)-u(2)
  fcn(14)4 : Fcn  Expr=(u(2)-u(3))/u(1)
  fcn(14)5 : Fcn  Expr=-u(2)/u(1)
  fcn1 : Fcn  Expr=u(2)+u(3)/u(1)
  fcn2 : Fcn  Expr=u(3)+(u(2)-u(3))*exp(-u(1)*u(4))
  Pt_new : Outport
  deco_stop_time : Outport  Port=2
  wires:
  In2/1 -> BS2/1
  Mem/1 -> Pt_new/1
  BS2/3 -> Mux2/4  "<stop_time>"
  fcn2/1 -> Mem/1
  Mux2/1 -> fcn2/1
  BS1/2 -> Mux2/2, Mux3/1  "<Pt_stop>"
  In1/1 -> BS1/1
  BS1/3 -> Mux4/1  "<He_b>"
  BS1/4 -> Mux4/2  "<M0>"
  Mux1/1 -> fcn(14)5/1
  BS1/1 -> Mux2/1, Mux1/1  "<He_k>"
  BS2/2 -> Mux2/3, Mux5/3, Mux3/2  "<Palv_next>"
  fcn1/1 -> Mux5/2  "M_next"
  fcn(14)5/1 -> deco_stop_time/1  "deco_stop_time"
  Mux4/1 -> fcn1/1
  >10e-320/1 -> fcn(14)1/1
  fcn(14)1/1 -> Mux1/2
  fcn(14)4/1 -> >10e-320/2, >10e-320/1
  Constant/1 -> >10e-320/3
  BS2/1 -> Mux4/3  "<Pstop_next>"
  Mux3/1 -> fcn(14)2/1
  fcn(14)2/1 -> >10e-300/1
  Mux5/1 -> fcn(14)4/1
  >10e-300/1 -> Mux5/1

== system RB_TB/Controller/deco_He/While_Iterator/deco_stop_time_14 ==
  note: Model: RB_TB/Controller/deco_He/While_Iterator/deco_stop_time_X
  In1 : Inport  Port=1  LatchInput=off
  In2 : Inport  Port=2  LatchInput=off
  >10e-300 : Saturate  UpperLimit=inf  LowerLimit=10e-320
  >10e-320 : Switch  Threshold=10e-320
  BS1 : BusSelector  DialogController=Simulink.DDGSource_Bus  OutputSignals=He_k,Pt_stop,He_b,M0
  BS2 : BusSelector  DialogController=Simulink.DDGSource_Bus  OutputSignals=Pstop_next,Palv_next,stop_time
  Constant : Constant
  Mem : Memory  InheritSampleTime=on
  Mux1 : Mux  Inputs=2
  Mux2 : Mux
  Mux3 : Mux  Inputs=2
  Mux4 : Mux  Inputs=3
  Mux5 : Mux  Inputs=3
  fcn(14)1 : Fcn  Expr=log(u(1))
  fcn(14)2 : Fcn  Expr=u(1)-u(2)
  fcn(14)4 : Fcn  Expr=(u(2)-u(3))/u(1)
  fcn(14)5 : Fcn  Expr=-u(2)/u(1)
  fcn1 : Fcn  Expr=u(2)+u(3)/u(1)
  fcn2 : Fcn  Expr=u(3)+(u(2)-u(3))*exp(-u(1)*u(4))
  Pt_new : Outport
  deco_stop_time : Outport  Port=2
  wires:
  >10e-300/1 -> Mux5/1
  Mux5/1 -> fcn(14)4/1
  fcn(14)2/1 -> >10e-300/1
  Mux3/1 -> fcn(14)2/1
  BS2/1 -> Mux4/3  "<Pstop_next>"
  Constant/1 -> >10e-320/3
  fcn(14)4/1 -> >10e-320/1, >10e-320/2
  fcn(14)1/1 -> Mux1/2
  >10e-320/1 -> fcn(14)1/1
  Mux4/1 -> fcn1/1
  fcn(14)5/1 -> deco_stop_time/1  "deco_stop_time"
  fcn1/1 -> Mux5/2  "M_next"
  BS2/2 -> Mux3/2, Mux5/3, Mux2/3  "<Palv_next>"
  BS1/1 -> Mux1/1, Mux2/1  "<He_k>"
  Mux1/1 -> fcn(14)5/1
  BS1/4 -> Mux4/2  "<M0>"
  BS1/3 -> Mux4/1  "<He_b>"
  In1/1 -> BS1/1
  BS1/2 -> Mux3/1, Mux2/2  "<Pt_stop>"
  Mux2/1 -> fcn2/1
  fcn2/1 -> Mem/1
  BS2/3 -> Mux2/4  "<stop_time>"
  Mem/1 -> Pt_new/1
  In2/1 -> BS2/1

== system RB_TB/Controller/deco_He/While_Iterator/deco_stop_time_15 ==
  note: Model: RB_TB/Controller/deco_He/While_Iterator/deco_stop_time_X
  In1 : Inport  Port=1  LatchInput=off
  In2 : Inport  Port=2  LatchInput=off
  >10e-300 : Saturate  UpperLimit=inf  LowerLimit=10e-320
  >10e-320 : Switch  Threshold=10e-320
  BS1 : BusSelector  DialogController=Simulink.DDGSource_Bus  OutputSignals=He_k,Pt_stop,He_b,M0
  BS2 : BusSelector  DialogController=Simulink.DDGSource_Bus  OutputSignals=Pstop_next,Palv_next,stop_time
  Constant : Constant
  Mem : Memory  InheritSampleTime=on
  Mux1 : Mux  Inputs=2
  Mux2 : Mux
  Mux3 : Mux  Inputs=2
  Mux4 : Mux  Inputs=3
  Mux5 : Mux  Inputs=3
  fcn(14)1 : Fcn  Expr=log(u(1))
  fcn(14)2 : Fcn  Expr=u(1)-u(2)
  fcn(14)4 : Fcn  Expr=(u(2)-u(3))/u(1)
  fcn(14)5 : Fcn  Expr=-u(2)/u(1)
  fcn1 : Fcn  Expr=u(2)+u(3)/u(1)
  fcn2 : Fcn  Expr=u(3)+(u(2)-u(3))*exp(-u(1)*u(4))
  Pt_new : Outport
  deco_stop_time : Outport  Port=2
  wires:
  In2/1 -> BS2/1
  Mem/1 -> Pt_new/1
  BS2/3 -> Mux2/4  "<stop_time>"
  fcn2/1 -> Mem/1
  Mux2/1 -> fcn2/1
  BS1/2 -> Mux2/2, Mux3/1  "<Pt_stop>"
  In1/1 -> BS1/1
  BS1/3 -> Mux4/1  "<He_b>"
  BS1/4 -> Mux4/2  "<M0>"
  Mux1/1 -> fcn(14)5/1
  BS1/1 -> Mux2/1, Mux1/1  "<He_k>"
  BS2/2 -> Mux2/3, Mux5/3, Mux3/2  "<Palv_next>"
  fcn1/1 -> Mux5/2  "M_next"
  fcn(14)5/1 -> deco_stop_time/1  "deco_stop_time"
  Mux4/1 -> fcn1/1
  >10e-320/1 -> fcn(14)1/1
  fcn(14)1/1 -> Mux1/2
  fcn(14)4/1 -> >10e-320/2, >10e-320/1
  Constant/1 -> >10e-320/3
  BS2/1 -> Mux4/3  "<Pstop_next>"
  Mux3/1 -> fcn(14)2/1
  fcn(14)2/1 -> >10e-300/1
  Mux5/1 -> fcn(14)4/1
  >10e-300/1 -> Mux5/1

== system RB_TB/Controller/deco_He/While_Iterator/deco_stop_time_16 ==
  note: Model: RB_TB/Controller/deco_He/While_Iterator/deco_stop_time_X
  In1 : Inport  Port=1  LatchInput=off
  In2 : Inport  Port=2  LatchInput=off
  >10e-300 : Saturate  UpperLimit=inf  LowerLimit=10e-320
  >10e-320 : Switch  Threshold=10e-320
  BS1 : BusSelector  DialogController=Simulink.DDGSource_Bus  OutputSignals=He_k,Pt_stop,He_b,M0
  BS2 : BusSelector  DialogController=Simulink.DDGSource_Bus  OutputSignals=Pstop_next,Palv_next,stop_time
  Constant : Constant
  Mem : Memory  InheritSampleTime=on
  Mux1 : Mux  Inputs=2
  Mux2 : Mux
  Mux3 : Mux  Inputs=2
  Mux4 : Mux  Inputs=3
  Mux5 : Mux  Inputs=3
  fcn(14)1 : Fcn  Expr=log(u(1))
  fcn(14)2 : Fcn  Expr=u(1)-u(2)
  fcn(14)4 : Fcn  Expr=(u(2)-u(3))/u(1)
  fcn(14)5 : Fcn  Expr=-u(2)/u(1)
  fcn1 : Fcn  Expr=u(2)+u(3)/u(1)
  fcn2 : Fcn  Expr=u(3)+(u(2)-u(3))*exp(-u(1)*u(4))
  Pt_new : Outport
  deco_stop_time : Outport  Port=2
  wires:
  >10e-300/1 -> Mux5/1
  Mux5/1 -> fcn(14)4/1
  fcn(14)2/1 -> >10e-300/1
  Mux3/1 -> fcn(14)2/1
  BS2/1 -> Mux4/3  "<Pstop_next>"
  Constant/1 -> >10e-320/3
  fcn(14)4/1 -> >10e-320/1, >10e-320/2
  fcn(14)1/1 -> Mux1/2
  >10e-320/1 -> fcn(14)1/1
  Mux4/1 -> fcn1/1
  fcn(14)5/1 -> deco_stop_time/1  "deco_stop_time"
  fcn1/1 -> Mux5/2  "M_next"
  BS2/2 -> Mux3/2, Mux5/3, Mux2/3  "<Palv_next>"
  BS1/1 -> Mux1/1, Mux2/1  "<He_k>"
  Mux1/1 -> fcn(14)5/1
  BS1/4 -> Mux4/2  "<M0>"
  BS1/3 -> Mux4/1  "<He_b>"
  In1/1 -> BS1/1
  BS1/2 -> Mux3/1, Mux2/2  "<Pt_stop>"
  Mux2/1 -> fcn2/1
  fcn2/1 -> Mem/1
  BS2/3 -> Mux2/4  "<stop_time>"
  Mem/1 -> Pt_new/1
  In2/1 -> BS2/1

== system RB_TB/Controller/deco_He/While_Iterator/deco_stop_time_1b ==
  note: Model: RB_TB/Controller/deco_He/While_Iterator/deco_stop_time_X
  In1 : Inport  Port=1  LatchInput=off
  In2 : Inport  Port=2  LatchInput=off
  >10e-300 : Saturate  UpperLimit=inf  LowerLimit=10e-320
  >10e-320 : Switch  Threshold=10e-320
  BS1 : BusSelector  DialogController=Simulink.DDGSource_Bus  OutputSignals=He_k,Pt_stop,He_b,M0
  BS2 : BusSelector  DialogController=Simulink.DDGSource_Bus  OutputSignals=Pstop_next,Palv_next,stop_time
  Constant : Constant
  Mem : Memory  InheritSampleTime=on
  Mux1 : Mux  Inputs=2
  Mux2 : Mux
  Mux3 : Mux  Inputs=2
  Mux4 : Mux  Inputs=3
  Mux5 : Mux  Inputs=3
  fcn(14)1 : Fcn  Expr=log(u(1))
  fcn(14)2 : Fcn  Expr=u(1)-u(2)
  fcn(14)4 : Fcn  Expr=(u(2)-u(3))/u(1)
  fcn(14)5 : Fcn  Expr=-u(2)/u(1)
  fcn1 : Fcn  Expr=u(2)+u(3)/u(1)
  fcn2 : Fcn  Expr=u(3)+(u(2)-u(3))*exp(-u(1)*u(4))
  Pt_new : Outport
  deco_stop_time : Outport  Port=2
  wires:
  >10e-300/1 -> Mux5/1
  Mux5/1 -> fcn(14)4/1
  fcn(14)2/1 -> >10e-300/1
  Mux3/1 -> fcn(14)2/1
  BS2/1 -> Mux4/3  "<Pstop_next>"
  Constant/1 -> >10e-320/3
  fcn(14)4/1 -> >10e-320/1, >10e-320/2
  fcn(14)1/1 -> Mux1/2
  >10e-320/1 -> fcn(14)1/1
  Mux4/1 -> fcn1/1
  fcn(14)5/1 -> deco_stop_time/1  "deco_stop_time"
  fcn1/1 -> Mux5/2  "M_next"
  BS2/2 -> Mux3/2, Mux5/3, Mux2/3  "<Palv_next>"
  BS1/1 -> Mux1/1, Mux2/1  "<He_k>"
  Mux1/1 -> fcn(14)5/1
  BS1/4 -> Mux4/2  "<M0>"
  BS1/3 -> Mux4/1  "<He_b>"
  In1/1 -> BS1/1
  BS1/2 -> Mux3/1, Mux2/2  "<Pt_stop>"
  Mux2/1 -> fcn2/1
  fcn2/1 -> Mem/1
  BS2/3 -> Mux2/4  "<stop_time>"
  Mem/1 -> Pt_new/1
  In2/1 -> BS2/1

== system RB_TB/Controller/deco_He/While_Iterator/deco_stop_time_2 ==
  note: Model: RB_TB/Controller/deco_He/While_Iterator/deco_stop_time_X
  In1 : Inport  Port=1  LatchInput=off
  In2 : Inport  Port=2  LatchInput=off
  >10e-300 : Saturate  UpperLimit=inf  LowerLimit=10e-320
  >10e-320 : Switch  Threshold=10e-320
  BS1 : BusSelector  DialogController=Simulink.DDGSource_Bus  OutputSignals=He_k,Pt_stop,He_b,M0
  BS2 : BusSelector  DialogController=Simulink.DDGSource_Bus  OutputSignals=Pstop_next,Palv_next,stop_time
  Constant : Constant
  Mem : Memory  InheritSampleTime=on
  Mux1 : Mux  Inputs=2
  Mux2 : Mux
  Mux3 : Mux  Inputs=2
  Mux4 : Mux  Inputs=3
  Mux5 : Mux  Inputs=3
  fcn(14)1 : Fcn  Expr=log(u(1))
  fcn(14)2 : Fcn  Expr=u(1)-u(2)
  fcn(14)4 : Fcn  Expr=(u(2)-u(3))/u(1)
  fcn(14)5 : Fcn  Expr=-u(2)/u(1)
  fcn1 : Fcn  Expr=u(2)+u(3)/u(1)
  fcn2 : Fcn  Expr=u(3)+(u(2)-u(3))*exp(-u(1)*u(4))
  Pt_new : Outport
  deco_stop_time : Outport  Port=2
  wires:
  In2/1 -> BS2/1
  Mem/1 -> Pt_new/1
  BS2/3 -> Mux2/4  "<stop_time>"
  fcn2/1 -> Mem/1
  Mux2/1 -> fcn2/1
  BS1/2 -> Mux2/2, Mux3/1  "<Pt_stop>"
  In1/1 -> BS1/1
  BS1/3 -> Mux4/1  "<He_b>"
  BS1/4 -> Mux4/2  "<M0>"
  Mux1/1 -> fcn(14)5/1
  BS1/1 -> Mux2/1, Mux1/1  "<He_k>"
  BS2/2 -> Mux2/3, Mux5/3, Mux3/2  "<Palv_next>"
  fcn1/1 -> Mux5/2  "M_next"
  fcn(14)5/1 -> deco_stop_time/1  "deco_stop_time"
  Mux4/1 -> fcn1/1
  >10e-320/1 -> fcn(14)1/1
  fcn(14)1/1 -> Mux1/2
  fcn(14)4/1 -> >10e-320/2, >10e-320/1
  Constant/1 -> >10e-320/3
  BS2/1 -> Mux4/3  "<Pstop_next>"
  Mux3/1 -> fcn(14)2/1
  fcn(14)2/1 -> >10e-300/1
  Mux5/1 -> fcn(14)4/1
  >10e-300/1 -> Mux5/1

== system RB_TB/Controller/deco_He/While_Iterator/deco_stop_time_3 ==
  note: Model: RB_TB/Controller/deco_He/While_Iterator/deco_stop_time_X
  In1 : Inport  Port=1  LatchInput=off
  In2 : Inport  Port=2  LatchInput=off
  >10e-300 : Saturate  UpperLimit=inf  LowerLimit=10e-320
  >10e-320 : Switch  Threshold=10e-320
  BS1 : BusSelector  DialogController=Simulink.DDGSource_Bus  OutputSignals=He_k,Pt_stop,He_b,M0
  BS2 : BusSelector  DialogController=Simulink.DDGSource_Bus  OutputSignals=Pstop_next,Palv_next,stop_time
  Constant : Constant
  Mem : Memory  InheritSampleTime=on
  Mux1 : Mux  Inputs=2
  Mux2 : Mux
  Mux3 : Mux  Inputs=2
  Mux4 : Mux  Inputs=3
  Mux5 : Mux  Inputs=3
  fcn(14)1 : Fcn  Expr=log(u(1))
  fcn(14)2 : Fcn  Expr=u(1)-u(2)
  fcn(14)4 : Fcn  Expr=(u(2)-u(3))/u(1)
  fcn(14)5 : Fcn  Expr=-u(2)/u(1)
  fcn1 : Fcn  Expr=u(2)+u(3)/u(1)
  fcn2 : Fcn  Expr=u(3)+(u(2)-u(3))*exp(-u(1)*u(4))
  Pt_new : Outport
  deco_stop_time : Outport  Port=2
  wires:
  In2/1 -> BS2/1
  Mem/1 -> Pt_new/1
  BS2/3 -> Mux2/4  "<stop_time>"
  fcn2/1 -> Mem/1
  Mux2/1 -> fcn2/1
  BS1/2 -> Mux2/2, Mux3/1  "<Pt_stop>"
  In1/1 -> BS1/1
  BS1/3 -> Mux4/1  "<He_b>"
  BS1/4 -> Mux4/2  "<M0>"
  Mux1/1 -> fcn(14)5/1
  BS1/1 -> Mux2/1, Mux1/1  "<He_k>"
  BS2/2 -> Mux2/3, Mux5/3, Mux3/2  "<Palv_next>"
  fcn1/1 -> Mux5/2  "M_next"
  fcn(14)5/1 -> deco_stop_time/1  "deco_stop_time"
  Mux4/1 -> fcn1/1
  >10e-320/1 -> fcn(14)1/1
  fcn(14)1/1 -> Mux1/2
  fcn(14)4/1 -> >10e-320/2, >10e-320/1
  Constant/1 -> >10e-320/3
  BS2/1 -> Mux4/3  "<Pstop_next>"
  Mux3/1 -> fcn(14)2/1
  fcn(14)2/1 -> >10e-300/1
  Mux5/1 -> fcn(14)4/1
  >10e-300/1 -> Mux5/1

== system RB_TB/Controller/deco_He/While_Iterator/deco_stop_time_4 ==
  note: Model: RB_TB/Controller/deco_He/While_Iterator/deco_stop_time_X
  In1 : Inport  Port=1  LatchInput=off
  In2 : Inport  Port=2  LatchInput=off
  >10e-300 : Saturate  UpperLimit=inf  LowerLimit=10e-320
  >10e-320 : Switch  Threshold=10e-320
  BS1 : BusSelector  DialogController=Simulink.DDGSource_Bus  OutputSignals=He_k,Pt_stop,He_b,M0
  BS2 : BusSelector  DialogController=Simulink.DDGSource_Bus  OutputSignals=Pstop_next,Palv_next,stop_time
  Constant : Constant
  Mem : Memory  InheritSampleTime=on
  Mux1 : Mux  Inputs=2
  Mux2 : Mux
  Mux3 : Mux  Inputs=2
  Mux4 : Mux  Inputs=3
  Mux5 : Mux  Inputs=3
  fcn(14)1 : Fcn  Expr=log(u(1))
  fcn(14)2 : Fcn  Expr=u(1)-u(2)
  fcn(14)4 : Fcn  Expr=(u(2)-u(3))/u(1)
  fcn(14)5 : Fcn  Expr=-u(2)/u(1)
  fcn1 : Fcn  Expr=u(2)+u(3)/u(1)
  fcn2 : Fcn  Expr=u(3)+(u(2)-u(3))*exp(-u(1)*u(4))
  Pt_new : Outport
  deco_stop_time : Outport  Port=2
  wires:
  >10e-300/1 -> Mux5/1
  Mux5/1 -> fcn(14)4/1
  fcn(14)2/1 -> >10e-300/1
  Mux3/1 -> fcn(14)2/1
  BS2/1 -> Mux4/3  "<Pstop_next>"
  Constant/1 -> >10e-320/3
  fcn(14)4/1 -> >10e-320/1, >10e-320/2
  fcn(14)1/1 -> Mux1/2
  >10e-320/1 -> fcn(14)1/1
  Mux4/1 -> fcn1/1
  fcn(14)5/1 -> deco_stop_time/1  "deco_stop_time"
  fcn1/1 -> Mux5/2  "M_next"
  BS2/2 -> Mux3/2, Mux5/3, Mux2/3  "<Palv_next>"
  BS1/1 -> Mux1/1, Mux2/1  "<He_k>"
  Mux1/1 -> fcn(14)5/1
  BS1/4 -> Mux4/2  "<M0>"
  BS1/3 -> Mux4/1  "<He_b>"
  In1/1 -> BS1/1
  BS1/2 -> Mux3/1, Mux2/2  "<Pt_stop>"
  Mux2/1 -> fcn2/1
  fcn2/1 -> Mem/1
  BS2/3 -> Mux2/4  "<stop_time>"
  Mem/1 -> Pt_new/1
  In2/1 -> BS2/1

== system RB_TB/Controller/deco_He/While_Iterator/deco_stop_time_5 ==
  note: Model: RB_TB/Controller/deco_He/While_Iterator/deco_stop_time_X
  In1 : Inport  Port=1  LatchInput=off
  In2 : Inport  Port=2  LatchInput=off
  >10e-300 : Saturate  UpperLimit=inf  LowerLimit=10e-320
  >10e-320 : Switch  Threshold=10e-320
  BS1 : BusSelector  DialogController=Simulink.DDGSource_Bus  OutputSignals=He_k,Pt_stop,He_b,M0
  BS2 : BusSelector  DialogController=Simulink.DDGSource_Bus  OutputSignals=Pstop_next,Palv_next,stop_time
  Constant : Constant
  Mem : Memory  InheritSampleTime=on
  Mux1 : Mux  Inputs=2
  Mux2 : Mux
  Mux3 : Mux  Inputs=2
  Mux4 : Mux  Inputs=3
  Mux5 : Mux  Inputs=3
  fcn(14)1 : Fcn  Expr=log(u(1))
  fcn(14)2 : Fcn  Expr=u(1)-u(2)
  fcn(14)4 : Fcn  Expr=(u(2)-u(3))/u(1)
  fcn(14)5 : Fcn  Expr=-u(2)/u(1)
  fcn1 : Fcn  Expr=u(2)+u(3)/u(1)
  fcn2 : Fcn  Expr=u(3)+(u(2)-u(3))*exp(-u(1)*u(4))
  Pt_new : Outport
  deco_stop_time : Outport  Port=2
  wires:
  In2/1 -> BS2/1
  Mem/1 -> Pt_new/1
  BS2/3 -> Mux2/4  "<stop_time>"
  fcn2/1 -> Mem/1
  Mux2/1 -> fcn2/1
  BS1/2 -> Mux2/2, Mux3/1  "<Pt_stop>"
  In1/1 -> BS1/1
  BS1/3 -> Mux4/1  "<He_b>"
  BS1/4 -> Mux4/2  "<M0>"
  Mux1/1 -> fcn(14)5/1
  BS1/1 -> Mux2/1, Mux1/1  "<He_k>"
  BS2/2 -> Mux2/3, Mux5/3, Mux3/2  "<Palv_next>"
  fcn1/1 -> Mux5/2  "M_next"
  fcn(14)5/1 -> deco_stop_time/1  "deco_stop_time"
  Mux4/1 -> fcn1/1
  >10e-320/1 -> fcn(14)1/1
  fcn(14)1/1 -> Mux1/2
  fcn(14)4/1 -> >10e-320/2, >10e-320/1
  Constant/1 -> >10e-320/3
  BS2/1 -> Mux4/3  "<Pstop_next>"
  Mux3/1 -> fcn(14)2/1
  fcn(14)2/1 -> >10e-300/1
  Mux5/1 -> fcn(14)4/1
  >10e-300/1 -> Mux5/1
